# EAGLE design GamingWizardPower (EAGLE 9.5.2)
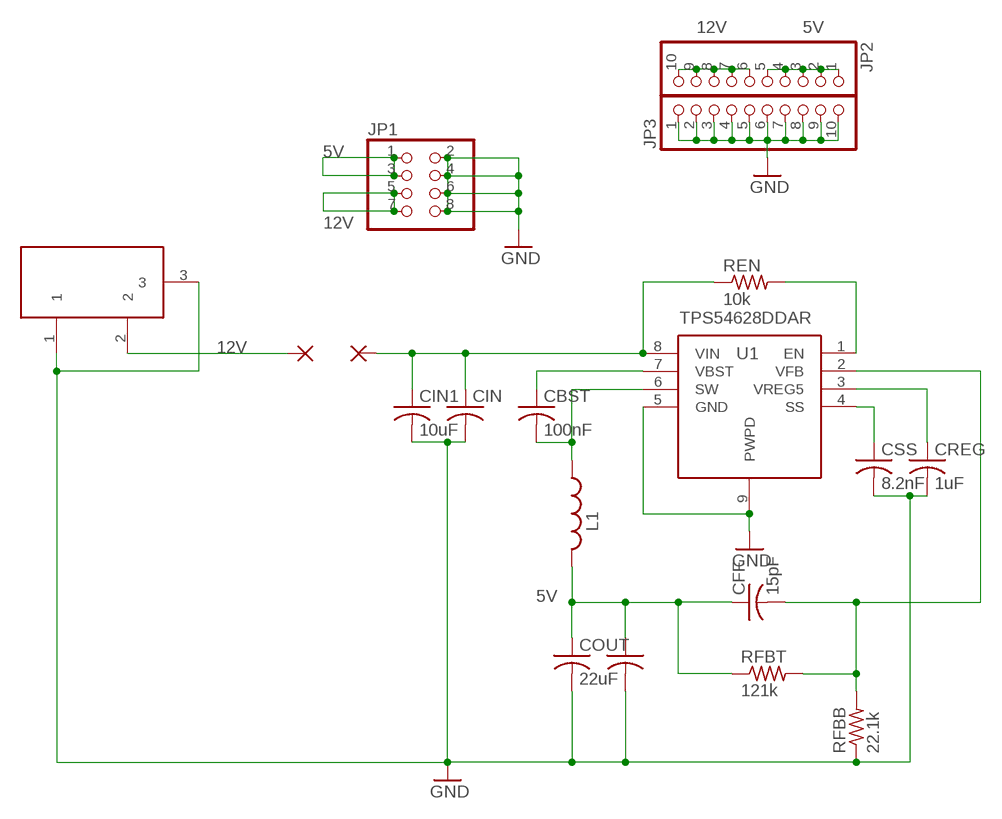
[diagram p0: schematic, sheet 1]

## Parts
CBST  100nF  C-USC0805  [C0805]
CFF  15pF  C-USC0805  [C0805]
CIN  10uF  C-USC1210K  [C1210K]
CIN1  10uF  C-USC1210K  [C1210K]
COUT  22uF  C-USC0805  [C0805]
COUT1  22uF  C-USC0805  [C0805]
CREG  1uF  C-USC0805  [C0805]
CSS  8.2nF  C-USC0805  [C0805]
JP1  PINHD-2X4  [2X04]
JP2  PINHD-1X10  [1X10]
JP3  PINHD-1X10  [1X10]
L1  3.3uH  HCM0703  [HCM0703]
PAD1  3,81/1,4  [3,81/1,4]
PAD2  3,81/1,4  [3,81/1,4]
REN  10k  R-US_R0805  [R0805]
RFBB  22.1k  R-US_R0805  [R0805]
RFBT  121k  R-US_R0805  [R0805]
U1  TPS54628DDAR  [SOIC127P600X170-9N]
X1  DC21MMX  [DC-21MM]

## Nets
5V: CFF.1 COUT1.1 COUT.1 JP1.1 JP1.3 JP2.1 JP2.2 JP2.3 JP2.4 JP2.5 L1.P$2 RFBT.1
12V: JP1.5 JP1.7 JP2.6 JP2.7 JP2.8 JP2.9 JP2.10 PAD1.1(P) X1.2
EN: REN.2 U1.1(EN)
GND: CIN1.2 CIN.2 COUT1.2 COUT.2 CREG.2 CSS.2 JP1.2 JP1.4 JP1.6 JP1.8 JP3.1 JP3.2 JP3.3 JP3.4 JP3.5 JP3.6 JP3.7 JP3.8 JP3.9 JP3.10 RFBB.1 U1.5(GND) U1.9(PWPD) X1.1 X1.3
SS: CSS.1 U1.4(SS)
SW: CBST.2 L1.P$1 U1.6(SW)
VBST: CBST.1 U1.7(VBST)
VFB: CFF.2 RFBB.2 RFBT.2 U1.2(VFB)
VIN: CIN1.1 CIN.1 PAD2.1(P) REN.1 U1.8(VIN)
VREG5: CREG.1 U1.3(VREG5)

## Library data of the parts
CBST = rcl:C-US: CAPACITOR, American symbol; MANUFACTURER: Samsung Electro-Mechanics; MANUFACTURER_PART_NUMBER: CL21F104ZBCNNNC; SPICEPREFIX: C
CFF = rcl:C-US: CAPACITOR, American symbol; MANUFACTURER: FH(Guangdong Fenghua Advanced Tech); MANUFACTURER_PART_NUMBER: 0805CG5R1C500NT; SPICEPREFIX: C
CIN CIN1 = rcl:C-US: CAPACITOR, American symbol; MANUFACTURER: Murata Electronics; MANUFACTURER_PART_NUMBER: GRM32ER71H106KA12L; SPICEPREFIX: C
COUT COUT1 = rcl:C-US: CAPACITOR, American symbol; MANUFACTURER: FH(Guangdong Fenghua Advanced Tech); MANUFACTURER_PART_NUMBER: 0805X226M160NT; SPICEPREFIX: C
CREG = rcl:C-US: CAPACITOR, American symbol; MANUFACTURER: Samsung Electro-Mechanics; MANUFACTURER_PART_NUMBER: CL21F105ZBFNNNE; SPICEPREFIX: C
CSS = rcl:C-US: CAPACITOR, American symbol; MANUFACTURER: Walsin Tech Corp; MANUFACTURER_PART_NUMBER: 0805B822K500CT; SPICEPREFIX: C
JP1 = pinhead:PINHD-2X4: PIN HEADER; MANUFACTURER: MINTRON; MANUFACTURER_PART_NUMBER: MTP125-1204S1
JP2 JP3 = pinhead:PINHD-1X10: PIN HEADER
L1 = HCM0703:HCM0703; MANUFACTURER: Eaton; MANUFACTURER_PART_NUMBER: HCM0703-3R3-R
PAD1 PAD2 = wirepad:3,81/1,4: THROUGH-HOLE PAD
REN = rcl:R-US_: RESISTOR, American symbol; MANUFACTURER: UNI-ROYAL(Uniroyal Elec); MANUFACTURER_PART_NUMBER: 0805W8F1002T5E; SPICEPREFIX: R
RFBB = rcl:R-US_: RESISTOR, American symbol; MANUFACTURER: UNI-ROYAL(Uniroyal Elec); MANUFACTURER_PART_NUMBER: 0805W8F2212T5E; SPICEPREFIX: R
RFBT = rcl:R-US_: RESISTOR, American symbol; MANUFACTURER: UNI-ROYAL(Uniroyal Elec); MANUFACTURER_PART_NUMBER: 0805W8F1213T5E; SPICEPREFIX: R
U1 = SamacSys_Parts:TPS54628DDAR: 4.5V to 18V Input, 6-A Synchronous Step-Down Converter with Eco-mode&#153; Source: Datasheet; DESCRIPTION: 4.5V to 18V Input, 6-A Synchronous Step-Down Converter with Eco-mode&#153;; HEIGHT: 1.7mm; MANUFACTURER_NAME: Texas Instruments; MANUFACTURER_PART_NUMBER: TPS54628DDAR; MOUSER_PART_NUMBER: 595-TPS54628DDAR; MOUSER_PRICE-STOCK: https://www.mouser.com/Search/Refine.aspx?Keyword=595-TPS54628DDAR
X1 = powersupply:DC21MM; MANUFACTURER: XKB Enterprise; MANUFACTURER_PART_NUMBER: DC-005-5A-2.0

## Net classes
0 default: width 0.508 mm, drill 0.508 mm, clearance 0.254 mm

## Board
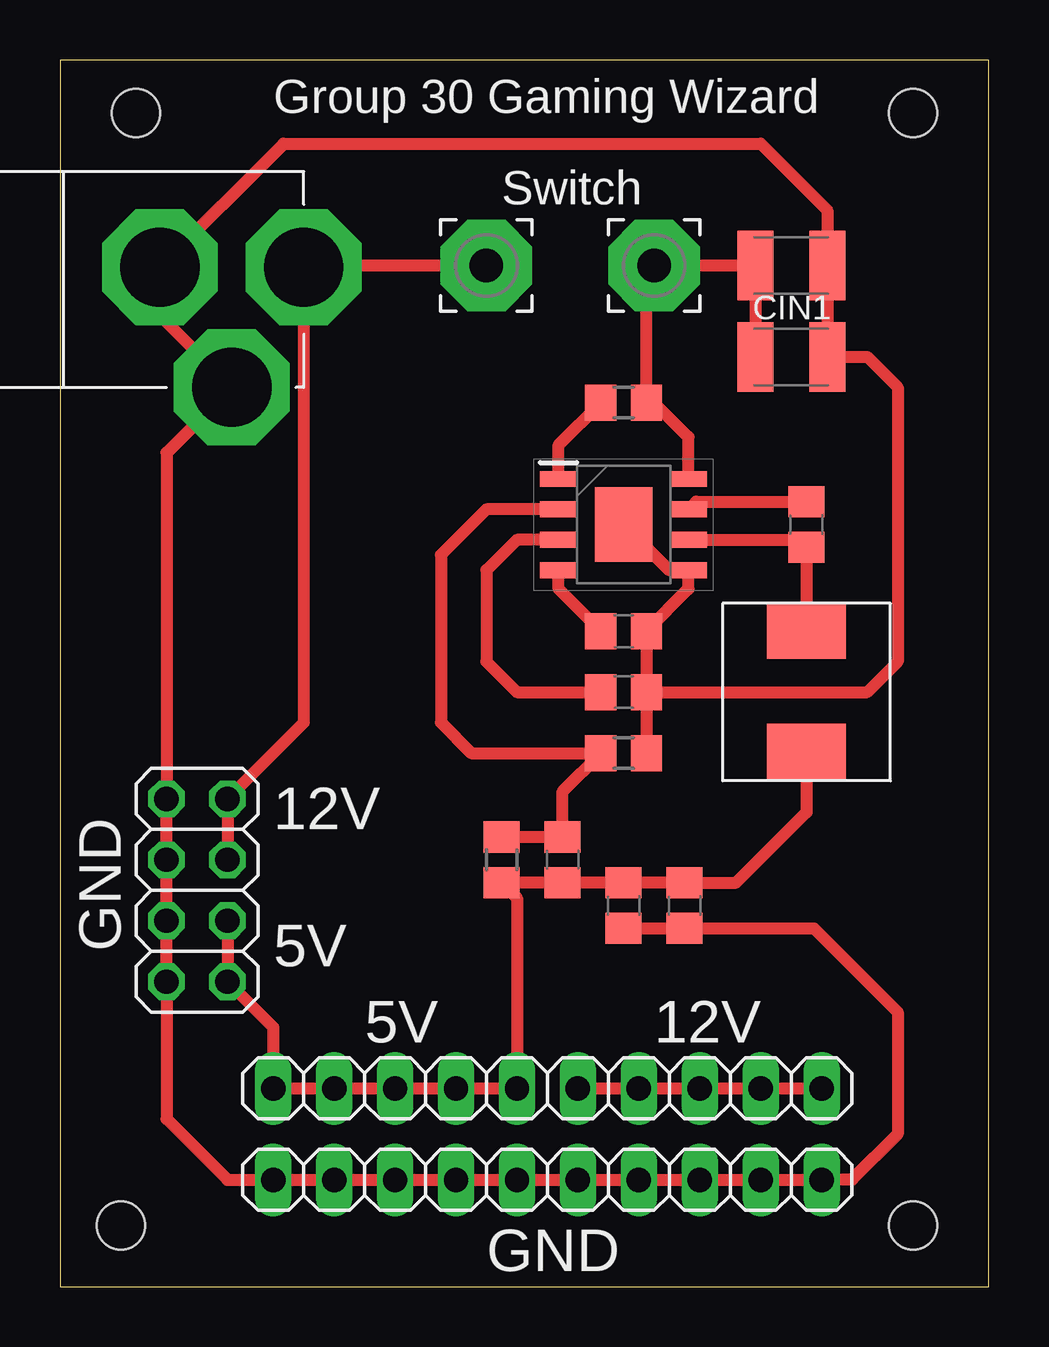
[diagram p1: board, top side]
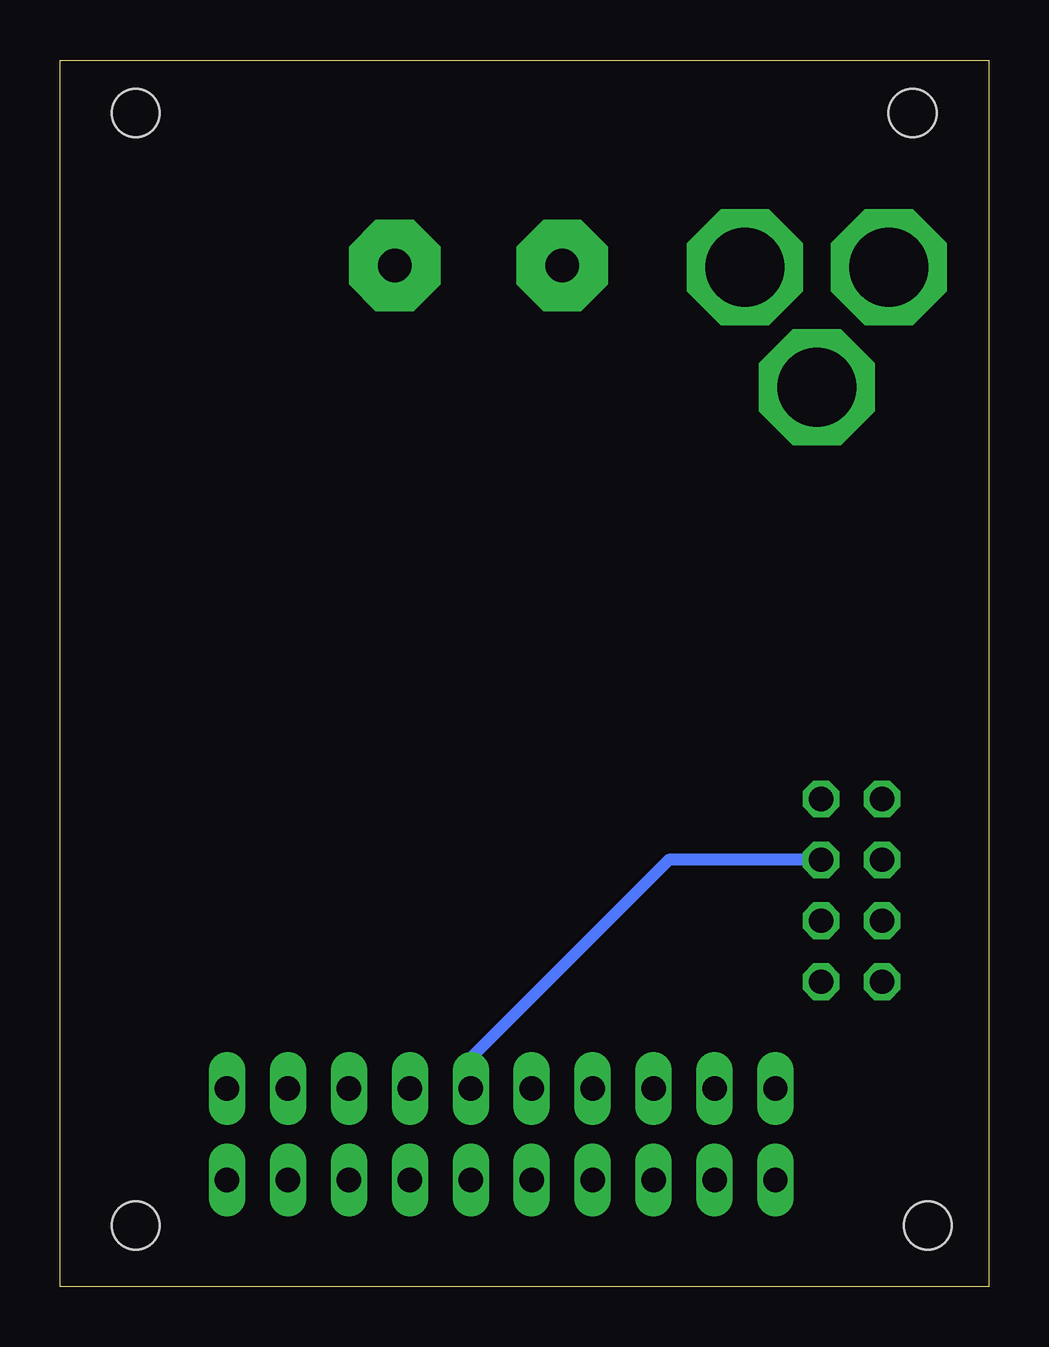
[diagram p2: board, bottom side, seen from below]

Size 38.72 x 51.1 mm. Coordinates in mm from the lower left corner, seen from the top.
Outline: 0,0 38.72,0 38.72,51.1 0,51.1 0,0
Copper layers (1*16): Top 0.035mm / dielectric 1.5mm / Bottom 0.035mm
Design rules "default": minimum track width 6mil, minimum drill 0.35mm, track to track 6mil, track to pad 6mil, pad to pad 6mil, via to via 6mil, smd to smd 6mil, copper to edge 40mil, drill to drill 6mil, minimum pad ring 10mil, minimum via ring 8mil, stop-mask expansion 4mil, vias tented up to drill 0mil, thermal gap 10mil
Holes 2 mm at 2.54,2.54 3.17,48.9 35.56,48.9 35.56,2.54

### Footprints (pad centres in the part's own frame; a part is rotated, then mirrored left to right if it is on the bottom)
C0805 = smd 1.3 x 1.5: 1 -0.95,0; 2 0.95,0
C1210K = smd 1.5 x 2.9: 1 -1.5,0; 2 1.5,0
2X04 = drill 1.016 octagon: 1 -3.81,-1.27; 2 -3.81,1.27; 3 -1.27,-1.27; 4 -1.27,1.27; 5 1.27,-1.27; 6 1.27,1.27; 7 3.81,-1.27; 8 3.81,1.27
1X10 = drill 1.016 long: 1 -11.43,0; 2 -8.89,0; 3 -6.35,0; 4 -3.81,0; 5 -1.27,0; 6 1.27,0; 7 3.81,0; 8 6.35,0; 9 8.89,0; 10 11.43,0
HCM0703 = smd 3.3 x 2.3: P$1 0,-2.54; P$2 0,2.47
3,81/1,4 = drill 1.397 pad 3.81 octagon: 1 0,0
R0805 = smd 1.3 x 1.5: 1 -0.95,0; 2 0.95,0
SOIC127P600X170-9N = smd 1.525 x 0.65: 1 -2.712,1.905; 2 -2.712,0.635; 3 -2.712,-0.635; 4 -2.712,-1.905; 5 2.712,-1.905; 6 2.712,-0.635; 7 2.712,0.635; 8 2.712,1.905 | smd 2.4 x 3.1: 9 0,0
DC-21MM = drill 3.302 pad 4.826 octagon: 1 -5.08,-3.353; 2 -0.076,-6.35; 3 -0.076,-0.356

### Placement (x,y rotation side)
CBST  31.11,31.75 270 top
CFF  20.95,17.78 90 top
CIN  30.48,42.55 0 top
CIN1  30.48,38.73 0 top
COUT  23.49,15.88 270 top
COUT1  26.04,15.88 270 top
CREG  23.49,24.77 0 top
CSS  23.49,27.3 0 top
JP1  5.71,16.51 90 top
JP2  20.32,8.26 0 top
JP3  20.32,4.45 0 top
L1  31.11,24.77 180 top
PAD1  17.78,42.55 0 top
PAD2  24.76,42.55 0 top
REN  23.49,36.83 180 top
RFBB  23.49,22.23 180 top
RFBT  18.41,17.78 90 top
U1  23.49,31.75 0 top
X1  3.81,42.55 90 top

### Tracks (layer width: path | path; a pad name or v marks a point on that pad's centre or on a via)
5V
  Top 0.508: L1.P$2 31.11,19.75 28.18,16.82 COUT1.1 COUT.1 CFF.1 RFBT.1 19.05,16.2 JP2.5 JP2.4 JP2.3 JP2.2 JP2.1 8.89,10.79 JP1.1 JP1.3
12V
  Top 0.508: PAD1.1 10.24,42.55 X1.2 10.16,23.5 JP1.7 JP1.5 | JP2.6 JP2.7 JP2.8 JP2.9 JP2.10
  Bottom 0.508: JP2.6 21.59,9.53 13.34,17.78 JP1.5
EN
  Top 0.508: U1.1 20.78,35.07 REN.2
GND
  Top 0.508: CIN1.2 CIN.2 31.98,44.85 29.21,47.62 9.32,47.62 X1.3 4.17,40.46 X1.1 4.45,34.75 JP1.8 JP1.6 JP1.4 JP1.2 4.45,6.99 6.99,4.45 JP3.1 JP3.2 JP3.3 JP3.4 JP3.5 JP3.6 JP3.7 JP3.8 JP3.9 JP3.10 33.02,4.45 34.93,6.35 34.93,11.43 31.43,14.93 COUT1.2 COUT.2 | 32.39,38.33 CIN1.2 | CREG.2 CSS.2 26.21,29.07 U1.5 25.4,29.84 U1.9 | CREG.2 RFBB.1 | CREG.2 33.66,24.77 34.93,26.04 34.93,37.47 33.66,38.73 CIN1.2
SS
  Top 0.508: CSS.1 20.78,29.07 U1.4
SW
  Top 0.508: U1.6 30.8,31.11 CBST.2 L1.P$1
VBST
  Top 0.508: U1.7 26.52,32.7 CBST.1
VFB
  Top 0.508: U1.2 17.78,32.38 15.88,30.48 15.88,23.5 17.14,22.23 RFBB.2 20.95,20.64 CFF.2 RFBT.2
VIN
  Top 0.152: 24.6,36.67 REN.1
  Top 0.508: 24.6,36.67 24.76,36.83 26.21,35.39 U1.8 | 28.57,38.33 CIN1.1 CIN.1 PAD2.1 24.44,42.23 REN.1
VREG5
  Top 0.508: U1.3 19.05,31.11 17.78,29.84 17.78,26.04 19.05,24.77 CREG.1

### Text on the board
tPlace: Group 30 Gaming Wizard | 12V | GND | 5V | 5V | 12V | GND
tNames: Switch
